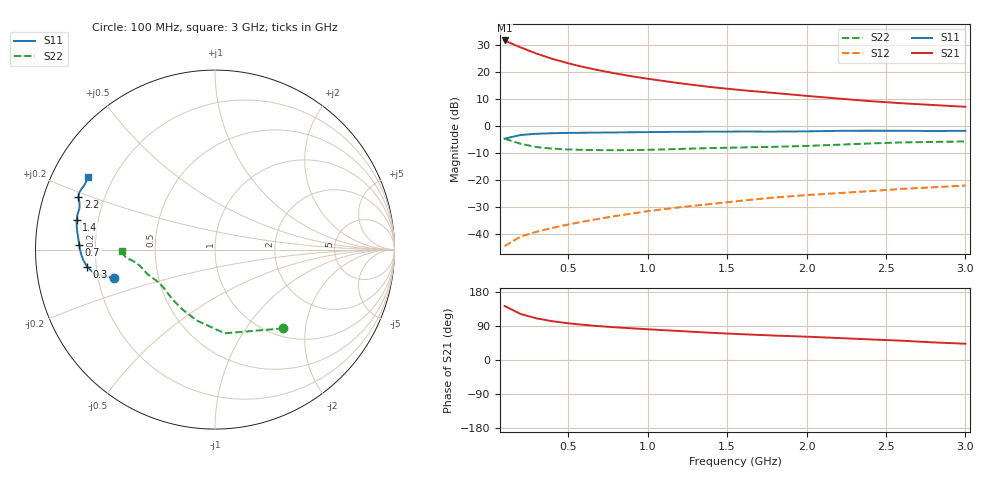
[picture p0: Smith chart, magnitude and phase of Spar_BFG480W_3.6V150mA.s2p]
! Filename: 3_6150BFG480.001
! Title: BFG480W
! Bias: Vce=3.6V; Ic=150mA
! Company: NXP Semiconductors NL
! User: Quality&Reliability T&D
! Measure time: 10 Nov 1999 / 12:02:00
#  MHz  S  MA  R 50
! Freq  S11  S21  S12  S22  :
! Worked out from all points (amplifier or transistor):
!   20 points, 100 MHz to 3 GHz, reference 50 ohm
!   highest |S21| = 31.8 dB at 100 MHz (marker M1)
!   |S21| within 3 dB of that: start of sweep to 219 MHz
!   unconditionally stable (mu >= 1): 375.8 MHz to end of sweep
!   at 400 MHz: K = 1.02, MAG = 30.6 dB, |S12| = -37.8 dB
!   at 1.2 GHz: K = 1.17, MAG = 20.6 dB, |S12| = -30.2 dB
!   at 3 GHz: K = 1.12, MAG = 12.5 dB, |S12| = -22.1 dB
!   S11 on the Smith chart (normalised r, x): 100 MHz: 0.27, -0.13; 300 MHz: 0.16, -0.06; 700 MHz: 0.14, +0.02; 1.4 GHz: 0.12, +0.10; 2.2 GHz: 0.11, +0.18; 3 GHz: 0.11, +0.26
100  0.5833 -164.1  38.82 142.5  0.005897 65.2  0.5815 -49.0
200  0.6826 -168.3  28.89 121.5  0.008865 59.6  0.4693 -83.4
300  0.719 -172.4  22.21 110.0  0.01089 60.5  0.4079 -104.4
400  0.7367 -175.5  17.68 102.4  0.01287 63.3  0.3803 -117.8
500  0.7464 -178.0  14.65 96.9  0.01489 65.7  0.3676 -127.0
600  0.7527 179.9  12.4 92.6  0.01695 68.0  0.361 -133.5
700  0.7566 178.0  10.76 89.2  0.01916 70.2  0.3574 -138.4
800  0.7616 176.2  9.45 86.2  0.02146 71.9  0.3565 -142.4
900  0.7667 174.6  8.401 83.6  0.02371 73.5  0.358 -145.9
1000  0.7722 173.0  7.566 81.1  0.02628 74.5  0.3621 -149.0
1200  0.7821 170.3  6.247 76.4  0.03104 75.9  0.3758 -154.0
1400  0.7881 168.0  5.288 71.8  0.03584 76.5  0.3906 -157.6
1600  0.7908 165.7  4.615 67.9  0.04139 77.0  0.4013 -160.5
1800  0.7893 163.2  4.106 64.5  0.04727 77.3  0.4124 -163.9
2000  0.7977 161.1  3.636 61.6  0.05223 77.8  0.4278 -167.8
2200  0.8146 159.1  3.242 58.0  0.05688 77.5  0.4502 -171.1
2400  0.8208 157.3  2.903 54.3  0.06188 76.9  0.4759 -173.3
2600  0.8167 155.5  2.651 50.9  0.06824 76.0  0.4967 -174.7
2800  0.8108 153.1  2.457 46.4  0.07303 74.4  0.5082 -176.5
3000  0.8161 150.4  2.282 43.0  0.07856 73.5  0.5179 -179.3
